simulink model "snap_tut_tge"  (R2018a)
settings: Solver=VariableStepDiscrete  StartTime=0.0  StopTime=50000  RelTol=1e-3
undefined symbols (not defined in the file): bad_frame, Bit, Both, bram, c, cnt_rst, core_rst, d, data, data_in, eof, eof_in, Falling, hex2dec, ip, ip_in, led, led_rx, led_tx, led_up, link_up, Location, Lower, Minimum_Area, notused, out, overrun, reg, Rising, ROACH2, sfp, SNAP, tx_full, tx_over, Unsigned, Upper, valid, valid_in, Width, xc7k160t
libraries: xbsIndex_r4 x1201, casper_library_misc x9, xps_library x5
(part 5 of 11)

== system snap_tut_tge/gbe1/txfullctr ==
  out_reg : Inport
  assert_reg : xbsIndex_r4/Assert  assert_type=on  type_source=Explicitly  gui_display_data_type=Fixed-point  arith_type=Unsigned  n_bits=32  bin_pt=0  preci_type=Single  exp_width=8  frac_width=24  assert_rate=off  rate_source=Explicitly  period=1  output_port=on  block_type=assert
  cast_gw : xbsIndex_r4/Convert  gui_display_data_type=Fixed-point  arith_type=Unsigned  n_bits=32  bin_pt=0  float_type=Single  exp_bits=8  fraction_bits=24  quantization=Truncate  overflow=Wrap  en=off  latency=1  pipeline=off  dbl_ovrd=off  block_type=convert
  io_delay : xbsIndex_r4/Delay  rst=off  infoeditControl=Selection of Reset will increase slice count due to use of real FFs and instead of SRLs  en=off  latency=1  reg_retiming=on  dbl_ovrd=off  block_type=delay
  reint1 : xbsIndex_r4/Reinterpret  force_arith_type=on  arith_type=Unsigned  force_bin_pt=on  bin_pt=0  block_type=reinterpret
  sim_out : Terminator
  snap_tut_tge_gbe1_txfullctr_user_data_in : xbsIndex_r4/Gateway Out  inherit_from_input=off  hdl_port=on  rows=1  columns=1  UseAsDAC=off  DACChannel='1'  interface=None  automatic_assignment=on  address_offset=hex2dec('00')  intf_name=''  intf_description=''  timing_constraint=None  locs_specified=off  LOCs={}  io_standard={}  block_type=gatewayout
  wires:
  io_delay/1 -> cast_gw/1
  cast_gw/1 -> snap_tut_tge_gbe1_txfullctr_user_data_in/1
  snap_tut_tge_gbe1_txfullctr_user_data_in/1 -> sim_out/1
  out_reg/1 -> assert_reg/1
  assert_reg/1 -> reint1/1
  reint1/1 -> io_delay/1

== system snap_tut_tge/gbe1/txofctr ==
  out_reg : Inport
  assert_reg : xbsIndex_r4/Assert  assert_type=on  type_source=Explicitly  gui_display_data_type=Fixed-point  arith_type=Unsigned  n_bits=32  bin_pt=0  preci_type=Single  exp_width=8  frac_width=24  assert_rate=off  rate_source=Explicitly  period=1  output_port=on  block_type=assert
  cast_gw : xbsIndex_r4/Convert  gui_display_data_type=Fixed-point  arith_type=Unsigned  n_bits=32  bin_pt=0  float_type=Single  exp_bits=8  fraction_bits=24  quantization=Truncate  overflow=Wrap  en=off  latency=1  pipeline=off  dbl_ovrd=off  block_type=convert
  io_delay : xbsIndex_r4/Delay  rst=off  infoeditControl=Selection of Reset will increase slice count due to use of real FFs and instead of SRLs  en=off  latency=1  reg_retiming=on  dbl_ovrd=off  block_type=delay
  reint1 : xbsIndex_r4/Reinterpret  force_arith_type=on  arith_type=Unsigned  force_bin_pt=on  bin_pt=0  block_type=reinterpret
  sim_out : Terminator
  snap_tut_tge_gbe1_txofctr_user_data_in : xbsIndex_r4/Gateway Out  inherit_from_input=off  hdl_port=on  rows=1  columns=1  UseAsDAC=off  DACChannel='1'  interface=None  automatic_assignment=on  address_offset=hex2dec('00')  intf_name=''  intf_description=''  timing_constraint=None  locs_specified=off  LOCs={}  io_standard={}  block_type=gatewayout
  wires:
  io_delay/1 -> cast_gw/1
  cast_gw/1 -> snap_tut_tge_gbe1_txofctr_user_data_in/1
  snap_tut_tge_gbe1_txofctr_user_data_in/1 -> sim_out/1
  out_reg/1 -> assert_reg/1
  assert_reg/1 -> reint1/1
  reint1/1 -> io_delay/1

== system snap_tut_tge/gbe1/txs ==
  in_link_up : Inport
  in_led_tx : Inport  Port=2
  in_tx_full : Inport  Port=3
  in_tx_over : Inport  Port=4
  in_valid : Inport  Port=5
  in_eof : Inport  Port=6
  in_data : Inport  Port=7
  in_ip : Inport  Port=8
  we : Inport  Port=9
  trig : Inport  Port=10
  assert_data : xbsIndex_r4/Assert  assert_type=on  type_source=Explicitly  gui_display_data_type=Fixed-point  arith_type=Unsigned  n_bits=64  bin_pt=0  preci_type=Single  exp_width=8  frac_width=24  assert_rate=off  rate_source=Explicitly  period=1  output_port=on  block_type=assert
  assert_eof : xbsIndex_r4/Assert  assert_type=on  type_source=Explicitly  gui_display_data_type=Boolean  arith_type=Boolean  n_bits=1  bin_pt=0  preci_type=Single  exp_width=8  frac_width=24  assert_rate=off  rate_source=Explicitly  period=1  output_port=on  block_type=assert
  assert_ip : xbsIndex_r4/Assert  assert_type=on  type_source=Explicitly  gui_display_data_type=Fixed-point  arith_type=Unsigned  n_bits=32  bin_pt=0  preci_type=Single  exp_width=8  frac_width=24  assert_rate=off  rate_source=Explicitly  period=1  output_port=on  block_type=assert
  assert_led_tx : xbsIndex_r4/Assert  assert_type=on  type_source=Explicitly  gui_display_data_type=Boolean  arith_type=Boolean  n_bits=1  bin_pt=0  preci_type=Single  exp_width=8  frac_width=24  assert_rate=off  rate_source=Explicitly  period=1  output_port=on  block_type=assert
  assert_link_up : xbsIndex_r4/Assert  assert_type=on  type_source=Explicitly  gui_display_data_type=Boolean  arith_type=Boolean  n_bits=1  bin_pt=0  preci_type=Single  exp_width=8  frac_width=24  assert_rate=off  rate_source=Explicitly  period=1  output_port=on  block_type=assert
  assert_tx_full : xbsIndex_r4/Assert  assert_type=on  type_source=Explicitly  gui_display_data_type=Boolean  arith_type=Boolean  n_bits=1  bin_pt=0  preci_type=Single  exp_width=8  frac_width=24  assert_rate=off  rate_source=Explicitly  period=1  output_port=on  block_type=assert
  assert_tx_over : xbsIndex_r4/Assert  assert_type=on  type_source=Explicitly  gui_display_data_type=Boolean  arith_type=Boolean  n_bits=1  bin_pt=0  preci_type=Single  exp_width=8  frac_width=24  assert_rate=off  rate_source=Explicitly  period=1  output_port=on  block_type=assert
  assert_valid : xbsIndex_r4/Assert  assert_type=on  type_source=Explicitly  gui_display_data_type=Boolean  arith_type=Boolean  n_bits=1  bin_pt=0  preci_type=Single  exp_width=8  frac_width=24  assert_rate=off  rate_source=Explicitly  period=1  output_port=on  block_type=assert
  buscreate : Subsystem  AncestorBlock=casper_library_flow_control/bus_create  mask(bus_create){inputNum=8}
      mask prompts: inputNum "Number of inputs:"
      mask init:
      | bus_create_init(gcb,...
      |     'inputNum', inputNum);
  io_delay : Subsystem  AncestorBlock=casper_library_delays/pipeline  mask(pipeline){csp_latency=5}
      mask prompts: csp_latency "Latency"
      mask help: An explicitly laid-out delay line to avoid mapping to SRL16s for use in pipelining to help achieve timing closure.
      mask init:
      | pipeline_init(gcb,'latency',csp_latency);
  ss : Subsystem  Tag=casper:snapshot  AncestorBlock=casper_library_scopes/snapshot  mask(snapshot){storage=bram, dram_dimm=2, dram_clock=250, nsamples=13, data_width=128, offset=off, circap=off, value=off, ext_arm=off, ext_circ=off, provide_outputs=off, use_dsp48=on}
      mask prompts: storage "Storage medium"; dram_dimm "DRAM dimm"; dram_clock "DRAM clock rate"; nsamples "Number of Samples (2^?)"; data_width "Data width"; offset "Start delay support"; circap "Circular capture support"; value "Extra value capture support"; ext_arm "External arm support"; ext_circ "External circular capture support"; provide_outputs "Provide outputs"; use_dsp48 "Use DSP48s to implement counters"
      mask help: Standard snap block, but with the following optional extras; 1) Optionally delay the fabric trigger by a user-specified number of valids. 2) Capture continuously after a trigger until a stop pulse is received. Data is captured into BRAM continuously, with old data being overwritten until a stop command is received. Then stop capturing when memory is filled. This enables you to get some data before and some data after the stop pulse. Use the 'tr_en_cnt' register to determine where you are in your vector. 'Addr' register's MSb now indicates 'busy capturing'. 3) Optionally capture a value on an i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
      mask init:
      | snapshot_init(gcb, ...
      |     'storage', storage, ...
      |     'dram_dimm', dram_dimm, ...
      |     'dram_clock', dram_clock, ...
      |     'nsamples', nsamples, ...
      |     'data_width', data_width, ...
      |     'offset', offset, ...
      |     'circap', circap, ...
      |     'value', value, ...
      |     'ext_arm', ext_arm, ...
      |     'ext_circ', ext_circ, ...
      |     'provide_outputs', 'off', ...
      |     'use_dsp48', use_dsp48);
  trig_delay : Subsystem  AncestorBlock=casper_library_delays/pipeline  mask(pipeline){csp_latency=5}
      mask prompts: csp_latency "Latency"
      mask help: An explicitly laid-out delay line to avoid mapping to SRL16s for use in pipelining to help achieve timing closure.
      mask init:
      | pipeline_init(gcb,'latency',csp_latency);
  we_delay : Subsystem  AncestorBlock=casper_library_delays/pipeline  mask(pipeline){csp_latency=5}
      mask prompts: csp_latency "Latency"
      mask help: An explicitly laid-out delay line to avoid mapping to SRL16s for use in pipelining to help achieve timing closure.
      mask init:
      | pipeline_init(gcb,'latency',csp_latency);
  arm_out : Outport
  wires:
  ss/1(arm_out) -> arm_out/1
  buscreate/1(bus_out) -> io_delay/1(d)
  io_delay/1(q) -> ss/1(din)
  in_link_up/1 -> assert_link_up/1
  assert_link_up/1 -> buscreate/1(in1)
  in_led_tx/1 -> assert_led_tx/1
  assert_led_tx/1 -> buscreate/2(in2)
  in_tx_full/1 -> assert_tx_full/1
  assert_tx_full/1 -> buscreate/3(in3)
  in_tx_over/1 -> assert_tx_over/1
  assert_tx_over/1 -> buscreate/4(in4)
  in_valid/1 -> assert_valid/1
  assert_valid/1 -> buscreate/5(in5)
  in_eof/1 -> assert_eof/1
  assert_eof/1 -> buscreate/6(in6)
  in_data/1 -> assert_data/1
  assert_data/1 -> buscreate/7(in7)
  in_ip/1 -> assert_ip/1
  assert_ip/1 -> buscreate/8(in8)
  we/1 -> we_delay/1(d)
  we_delay/1(q) -> ss/2(we)
  trig/1 -> trig_delay/1(d)
  trig_delay/1(q) -> ss/3(trig)

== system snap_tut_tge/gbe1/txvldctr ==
  out_reg : Inport
  assert_reg : xbsIndex_r4/Assert  assert_type=on  type_source=Explicitly  gui_display_data_type=Fixed-point  arith_type=Unsigned  n_bits=32  bin_pt=0  preci_type=Single  exp_width=8  frac_width=24  assert_rate=off  rate_source=Explicitly  period=1  output_port=on  block_type=assert
  cast_gw : xbsIndex_r4/Convert  gui_display_data_type=Fixed-point  arith_type=Unsigned  n_bits=32  bin_pt=0  float_type=Single  exp_bits=8  fraction_bits=24  quantization=Truncate  overflow=Wrap  en=off  latency=1  pipeline=off  dbl_ovrd=off  block_type=convert
  io_delay : xbsIndex_r4/Delay  rst=off  infoeditControl=Selection of Reset will increase slice count due to use of real FFs and instead of SRLs  en=off  latency=1  reg_retiming=on  dbl_ovrd=off  block_type=delay
  reint1 : xbsIndex_r4/Reinterpret  force_arith_type=on  arith_type=Unsigned  force_bin_pt=on  bin_pt=0  block_type=reinterpret
  sim_out : Terminator
  snap_tut_tge_gbe1_txvldctr_user_data_in : xbsIndex_r4/Gateway Out  inherit_from_input=off  hdl_port=on  rows=1  columns=1  UseAsDAC=off  DACChannel='1'  interface=None  automatic_assignment=on  address_offset=hex2dec('00')  intf_name=''  intf_description=''  timing_constraint=None  locs_specified=off  LOCs={}  io_standard={}  block_type=gatewayout
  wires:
  io_delay/1 -> cast_gw/1
  cast_gw/1 -> snap_tut_tge_gbe1_txvldctr_user_data_in/1
  snap_tut_tge_gbe1_txvldctr_user_data_in/1 -> sim_out/1
  out_reg/1 -> assert_reg/1
  assert_reg/1 -> reint1/1
  reint1/1 -> io_delay/1

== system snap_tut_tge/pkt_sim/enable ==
  sim_1 : Inport
  convert1_1 : DataTypeConversion  OutDataTypeStr=fixdt('ufix32_En0')
  convert2_1 : DataTypeConversion  OutDataTypeStr=fixdt('ufix32_En0')  ConvertRealWorld=Stored Integer (SI)
  gain_1 : Gain
  io_delay : xbsIndex_r4/Delay  rst=off  infoeditControl=Selection of Reset will increase slice count due to use of real FFs and instead of SRLs  en=off  latency=0  reg_retiming=on  dbl_ovrd=off  block_type=delay
  reint1 : xbsIndex_r4/Reinterpret  force_arith_type=on  arith_type=Unsigned  force_bin_pt=on  bin_pt=0  block_type=reinterpret
  slice_reg : xbsIndex_r4/Slice  nbits=32  boolean_output=off  mode=Lower Bit Location + Width  bit1=0  base1=MSB of Input  bit0=0  base0=LSB of Input  dbl_ovrd=off  block_type=slice
  snap_tut_tge_pkt_sim_enable_user_data_out : xbsIndex_r4/Gateway In  gui_display_data_type=Fixed-point  arith_type=Unsigned  n_bits=32  bin_pt=0  preci_type=Single  exp_width=8  frac_width=24  rows=1  columns=1  quantization="Round  (unbiased: +/- Inf)"  overflow=Saturate  period=1  UseAsADC=off  ADCChannel='1'  interface=None  automatic_assignment=on  address_offset=hex2dec('00')  intf_name=''  intf_description=''  default_value=0  timing_constraint=None  locs_specified=off  LOCs={}  io_standard={}  inherit_from_input=off  hdl_port=on  dbl_ovrd=off  block_type=gatewayin
  in_reg : Outport
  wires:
  snap_tut_tge_pkt_sim_enable_user_data_out/1 -> io_delay/1
  sim_1/1 -> convert1_1/1
  convert1_1/1 -> convert2_1/1
  convert2_1/1 -> gain_1/1
  gain_1/1 -> snap_tut_tge_pkt_sim_enable_user_data_out/1
  io_delay/1 -> slice_reg/1
  slice_reg/1 -> reint1/1
  reint1/1 -> in_reg/1

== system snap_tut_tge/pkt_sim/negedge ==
  in : Inport
  Delay : xbsIndex_r4/Delay  rst=off  infoeditControl=Selection of Reset will increase slice count due to use of real FFs and instead of SRLs  en=off  latency=1  reg_retiming=off  dbl_ovrd=off  block_type=delay
  Inverter : xbsIndex_r4/Inverter  en=off  latency=0  dbl_ovrd=off  block_type=inv
  edge_op : xbsIndex_r4/Logical  logical_function=AND  inputs=2  en=off  latency=0  precision=Full  arith_type=Unsigned  n_bits=8  bin_pt=2  align_bp=on  dbl_ovrd=off  block_type=logical
  out : Outport
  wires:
  Inverter/1 -> edge_op/1
  edge_op/1 -> out/1
  in/1 -> Inverter/1, Delay/1
  Delay/1 -> edge_op/2

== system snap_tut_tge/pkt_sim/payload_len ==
  sim_1 : Inport
  convert1_1 : DataTypeConversion  OutDataTypeStr=fixdt('ufix32_En0')
  convert2_1 : DataTypeConversion  OutDataTypeStr=fixdt('ufix32_En0')  ConvertRealWorld=Stored Integer (SI)
  gain_1 : Gain
  io_delay : xbsIndex_r4/Delay  rst=off  infoeditControl=Selection of Reset will increase slice count due to use of real FFs and instead of SRLs  en=off  latency=0  reg_retiming=on  dbl_ovrd=off  block_type=delay
  reint1 : xbsIndex_r4/Reinterpret  force_arith_type=on  arith_type=Unsigned  force_bin_pt=on  bin_pt=0  block_type=reinterpret
  slice_reg : xbsIndex_r4/Slice  nbits=32  boolean_output=off  mode=Lower Bit Location + Width  bit1=0  base1=MSB of Input  bit0=0  base0=LSB of Input  dbl_ovrd=off  block_type=slice
  snap_tut_tge_pkt_sim_payload_len_user_data_out : xbsIndex_r4/Gateway In  gui_display_data_type=Fixed-point  arith_type=Unsigned  n_bits=32  bin_pt=0  preci_type=Single  exp_width=8  frac_width=24  rows=1  columns=1  quantization="Round  (unbiased: +/- Inf)"  overflow=Saturate  period=1  UseAsADC=off  ADCChannel='1'  interface=None  automatic_assignment=on  address_offset=hex2dec('00')  intf_name=''  intf_description=''  default_value=0  timing_constraint=None  locs_specified=off  LOCs={}  io_standard={}  inherit_from_input=off  hdl_port=on  dbl_ovrd=off  block_type=gatewayin
  in_reg : Outport
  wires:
  snap_tut_tge_pkt_sim_payload_len_user_data_out/1 -> io_delay/1
  sim_1/1 -> convert1_1/1
  convert1_1/1 -> convert2_1/1
  convert2_1/1 -> gain_1/1
  gain_1/1 -> snap_tut_tge_pkt_sim_payload_len_user_data_out/1
  io_delay/1 -> slice_reg/1
  slice_reg/1 -> reint1/1
  reint1/1 -> in_reg/1

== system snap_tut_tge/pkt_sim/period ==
  sim_1 : Inport
  convert1_1 : DataTypeConversion  OutDataTypeStr=fixdt('ufix32_En0')
  convert2_1 : DataTypeConversion  OutDataTypeStr=fixdt('ufix32_En0')  ConvertRealWorld=Stored Integer (SI)
  gain_1 : Gain
  io_delay : xbsIndex_r4/Delay  rst=off  infoeditControl=Selection of Reset will increase slice count due to use of real FFs and instead of SRLs  en=off  latency=0  reg_retiming=on  dbl_ovrd=off  block_type=delay
  reint1 : xbsIndex_r4/Reinterpret  force_arith_type=on  arith_type=Unsigned  force_bin_pt=on  bin_pt=0  block_type=reinterpret
  slice_reg : xbsIndex_r4/Slice  nbits=32  boolean_output=off  mode=Lower Bit Location + Width  bit1=0  base1=MSB of Input  bit0=0  base0=LSB of Input  dbl_ovrd=off  block_type=slice
  snap_tut_tge_pkt_sim_period_user_data_out : xbsIndex_r4/Gateway In  gui_display_data_type=Fixed-point  arith_type=Unsigned  n_bits=32  bin_pt=0  preci_type=Single  exp_width=8  frac_width=24  rows=1  columns=1  quantization="Round  (unbiased: +/- Inf)"  overflow=Saturate  period=1  UseAsADC=off  ADCChannel='1'  interface=None  automatic_assignment=on  address_offset=hex2dec('00')  intf_name=''  intf_description=''  default_value=0  timing_constraint=None  locs_specified=off  LOCs={}  io_standard={}  inherit_from_input=off  hdl_port=on  dbl_ovrd=off  block_type=gatewayin
  in_reg : Outport
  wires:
  snap_tut_tge_pkt_sim_period_user_data_out/1 -> io_delay/1
  sim_1/1 -> convert1_1/1
  convert1_1/1 -> convert2_1/1
  convert2_1/1 -> gain_1/1
  gain_1/1 -> snap_tut_tge_pkt_sim_period_user_data_out/1
  io_delay/1 -> slice_reg/1
  slice_reg/1 -> reint1/1
  reint1/1 -> in_reg/1

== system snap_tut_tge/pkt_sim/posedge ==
  in : Inport
  Delay : xbsIndex_r4/Delay  rst=off  infoeditControl=Selection of Reset will increase slice count due to use of real FFs and instead of SRLs  en=off  latency=1  reg_retiming=off  dbl_ovrd=off  block_type=delay
  Inverter : xbsIndex_r4/Inverter  en=off  latency=0  dbl_ovrd=off  block_type=inv
  edge_op : xbsIndex_r4/Logical  logical_function=NOR  inputs=2  en=off  latency=0  precision=Full  arith_type=Unsigned  n_bits=8  bin_pt=2  align_bp=on  dbl_ovrd=off  block_type=logical
  out : Outport
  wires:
  Inverter/1 -> edge_op/1
  edge_op/1 -> out/1
  in/1 -> Inverter/1, Delay/1
  Delay/1 -> edge_op/2

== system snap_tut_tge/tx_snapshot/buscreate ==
  in1 : Inport
  in2 : Inport  Port=2
  in3 : Inport  Port=3
  concatenate : xbsIndex_r4/Concat  num_inputs=3  dbl_ovrd=off  block_type=concat
  reinterpret1 : xbsIndex_r4/Reinterpret  force_arith_type=on  arith_type=Unsigned  force_bin_pt=on  bin_pt=0  block_type=reinterpret
  reinterpret2 : xbsIndex_r4/Reinterpret  force_arith_type=on  arith_type=Unsigned  force_bin_pt=on  bin_pt=0  block_type=reinterpret
  reinterpret3 : xbsIndex_r4/Reinterpret  force_arith_type=on  arith_type=Unsigned  force_bin_pt=on  bin_pt=0  block_type=reinterpret
  bus_out : Outport
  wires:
  concatenate/1 -> bus_out/1
  in1/1 -> reinterpret1/1
  reinterpret1/1 -> concatenate/1
  in2/1 -> reinterpret2/1
  reinterpret2/1 -> concatenate/2
  in3/1 -> reinterpret3/1
  reinterpret3/1 -> concatenate/3

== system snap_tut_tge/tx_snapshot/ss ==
  note: Generate stop when in circular capture mode
  note: Delay start of capture
  note: ctrl: bit0: Put a posedge here to enable a new capture. bit1: ignore external trigger and trigger immediately. bit2: ignore external write enable and capture on every FPGA clock. bit3: continuously capture data until we get an external stop command.
  note: Offset in vector from first element captured, used during circular capture
  note: Number of bytes in buffer and done bit
  note: Number of valid data samples to skip after trigger before starting capture
  note: Value on vin aligned with first sample on din captured
  din : Inport
  we : Inport  Port=2
  trig : Inport  Port=3
  add_del : xbsIndex_r4/Delay  rst=off  infoeditControl=Selection of Reset will increase slice count due to use of real FFs and instead of SRLs  en=off  latency=1  reg_retiming=on  dbl_ovrd=off  block_type=delay
  add_gen : Subsystem  AncestorBlock=casper_library_scopes/snapshot/add_gen  mask{counter_size=12+4+1, increment=16, nsamples=12, burst_size=0, use_dsp48=on}
      mask prompts: counter_size "Address counter size (2^?)"; increment "Address counter increment"; nsamples "Number of samples (2^?)"; burst_size "Burst size (2^?)"; use_dsp48 "dsp48 counter/s"
      mask init:
      | set_param(gcb,'LinkStatus','inactive');
      | if strcmp(use_dsp48,'on'),
      |     set_param([gcb,'/add_gen'],'implementation','DSP48');
      | else
      |     set_param([gcb,'/add_gen'],'implementation','Fabric');
      | end
  arm : xbsIndex_r4/Constant  const=0  gui_display_data_type=Fixed-point  arith_type=Boolean  n_bits=16  bin_pt=14  preci_type=Single  exp_width=8  frac_width=24  explicit_period=on  period=1  equ=P=C  opselect=C  inp2=PCIN>>17  opr=+  inp1=P  carry=CIN  dbl_ovrd=off  block_type=constant
  arm_or : xbsIndex_r4/Logical  logical_function=OR  inputs=2  en=off  latency=0  precision=Full  arith_type=Unsigned  n_bits=16  bin_pt=0  align_bp=on  dbl_ovrd=off  block_type=logical
  basic_ctrl : Subsystem  AncestorBlock=casper_library_scopes/snapshot/basic_ctrl  mask{dram=off, data_width=128}
      mask prompts: data_width "data width"
      mask init:
      | set_param(gcb,'LinkStatus','inactive');
      | set_param([gcb,'/dram_munge'], 'dram', dram);
  bram : Subsystem  Tag=xps:bram  AncestorBlock=xps_library/Memory/shared_bram  mask{arith_type=Unsigned, addr_width=12, data_width=128, reg_prim_output=off, reg_core_output=off, optimization=Minimum_Area, data_bin_pt=0, init_vals=[0:2^12-1], sample_rate=1}
      mask prompts: arith_type "Output Data Type"; addr_width "Address width"; data_width "Data Width"; reg_prim_output "Register Primitive Output"; reg_core_output "Register Core Output"; data_bin_pt "Data Binary Point"; init_vals "Initial values (simulation only)"; sample_rate "Sample rate"
      mask init:
      | shared_bram_mask;
  cast : xbsIndex_r4/Convert  gui_display_data_type=Fixed-point  arith_type=Unsigned  n_bits=128  bin_pt=0  float_type=Single  exp_bits=8  fraction_bits=24  quantization=Truncate  overflow=Wrap  en=off  latency=0  pipeline=off  dbl_ovrd=off  block_type=convert
  circ : xbsIndex_r4/Constant  const=0  gui_display_data_type=Fixed-point  arith_type=Boolean  n_bits=16  bin_pt=14  preci_type=Single  exp_width=8  frac_width=24  explicit_period=on  period=1  equ=P=C  opselect=C  inp2=PCIN>>17  opr=+  inp1=P  carry=CIN  dbl_ovrd=off  block_type=constant
  circ_or : xbsIndex_r4/Logical  logical_function=OR  inputs=2  en=off  latency=0  precision=Full  arith_type=Unsigned  n_bits=16  bin_pt=0  align_bp=on  dbl_ovrd=off  block_type=logical
  ctrl : Subsystem  Tag=xps:sw_reg  AncestorBlock=xps_library/Memory/software_register  mask(swreg){io_dir=From Processor, io_delay=0, init_val=0, sample_period=1, names=reg, bitwidths=32, bin_pts=0, arith_types=0, sim_port=off, show_format=on}
      mask prompts: io_dir "I/O direction"; io_delay "I/O delay"; init_val "Initial Value"; sample_period "Sample period"; names "Bitfield names [msb...lsb]"; bitwidths "Bitfield widths"; bin_pts "Bitfield binary pts"; arith_types "Bitfield types, ufix=0, fix=1, bool=2"; sim_port "Provide sim input/output?"; show_format "Print format string?"
      mask help: A 32-bit software-accessible register. Can be divided into bitfields of varying widths and types using the fields in the block mask.
      mask init:
      | swreg_init(gcb)
  ctrl_combine : Subsystem  AncestorBlock=casper_library_flow_control/bus_create  mask(bus_create){inputNum=4}
      mask prompts: inputNum "Number of inputs:"
      mask init:
      | bus_create_init(gcb,...
      |     'inputNum', inputNum);
  ctrl_split : Subsystem  AncestorBlock=casper_library_flow_control/bus_expand  mask(bus_expand){mode=divisions of arbitrary size, outputNum=1, outputWidth=[28 1 2 1], outputBinaryPt=0, outputArithmeticType=[0 2 0 2], show_format=on, outputToWorkspace=off, variablePrefix=out, outputToModelAsWell=on}
      mask prompts: outputNum "Number of outputs:"; outputWidth "Output width [msb ... lsb]:"; outputBinaryPt "Output binary point position [msb ... lsb]:"; outputArithmeticType "Output arithmetic type (ufix=0, fix=1, bool=2) [msb ... lsb]:"; show_format "Print format string?"; outputToWorkspace "Output to workspace?"; variablePrefix "Variable name prefix:"; outputToModelAsWell "Output to model as well?"
      mask help: Expands a 'bus' made using a bus_create or Xilinx concat block. The input will be divided into the specified number of outputs with the specified arithmetic types. Divisions are made from most significant bit.
      mask init:
      | bus_expand_init(gcb,...
      |     'mode', mode, ...
      |     'outputNum', outputNum, ...
      |     'outputWidth', outputWidth, ...
      |     'outputBinaryPt', outputBinaryPt, ...
      |     'outputArithmeticType', outputArithmeticType, ...
      |     'show_format', show_format, ...
      |     'outputToWorkspace', outputToWorkspace, ...
      |     'variablePrefix', variablePrefix, ...
      |     'outputToModelAsWell', outputToModelAsWell);
  dat_del : xbsIndex_r4/Delay  rst=off  infoeditControl=Selection of Reset will increase slice count due to use of real FFs and instead of SRLs  en=off  latency=1  reg_retiming=on  dbl_ovrd=off  block_type=delay
  g_tr_en_cnt : Terminator
  gbram : Terminator
  goto_ss_we2_const : xbsIndex_r4/Constant  const=0  gui_display_data_type=Fixed-point  arith_type=Boolean  n_bits=16  bin_pt=14  preci_type=Single  exp_width=8  frac_width=24  explicit_period=on  period=1  equ=P=C  opselect=C  inp2=PCIN>>17  opr=+  inp1=P  carry=CIN  dbl_ovrd=off  block_type=constant
  goto_ss_we3_const : xbsIndex_r4/Constant  const=0  gui_display_data_type=Fixed-point  arith_type=Boolean  n_bits=16  bin_pt=14  preci_type=Single  exp_width=8  frac_width=24  explicit_period=on  period=1  equ=P=C  opselect=C  inp2=PCIN>>17  opr=+  inp1=P  carry=CIN  dbl_ovrd=off  block_type=constant
  gval : Terminator
  never : xbsIndex_r4/Constant  const=0  gui_display_data_type=Fixed-point  arith_type=Boolean  n_bits=16  bin_pt=14  preci_type=Single  exp_width=8  frac_width=24  explicit_period=on  period=1  equ=P=C  opselect=C  inp2=PCIN>>17  opr=+  inp1=P  carry=CIN  dbl_ovrd=off  block_type=constant
  ri : xbsIndex_r4/Reinterpret  force_arith_type=on  arith_type=Unsigned  force_bin_pt=on  bin_pt=0  block_type=reinterpret
  status : Subsystem  Tag=xps:sw_reg  AncestorBlock=xps_library/Memory/software_register  mask(swreg){io_dir=To Processor, io_delay=0, init_val=0, sample_period=1, names=reg, bitwidths=32, bin_pts=0, arith_types=0, sim_port=off, show_format=on}
      mask prompts: io_dir "I/O direction"; io_delay "I/O delay"; init_val "Initial Value"; sample_period "Sample period"; names "Bitfield names [msb...lsb]"; bitwidths "Bitfield widths"; bin_pts "Bitfield binary pts"; arith_types "Bitfield types, ufix=0, fix=1, bool=2"; sim_port "Provide sim input/output?"; show_format "Print format string?"
      mask help: A 32-bit software-accessible register. Can be divided into bitfields of varying widths and types using the fields in the block mask.
      mask init:
      | swreg_init(gcb)
  vin_const : xbsIndex_r4/Constant  const=0  gui_display_data_type=Fixed-point  arith_type=Boolean  n_bits=16  bin_pt=14  preci_type=Single  exp_width=8  frac_width=24  explicit_period=on  period=1  equ=P=C  opselect=C  inp2=PCIN>>17  opr=+  inp1=P  carry=CIN  dbl_ovrd=off  block_type=constant
  we_del : xbsIndex_r4/Delay  rst=off  infoeditControl=Selection of Reset will increase slice count due to use of real FFs and instead of SRLs  en=off  latency=1  reg_retiming=on  dbl_ovrd=off  block_type=delay
  arm_out : Outport
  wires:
  din/1 -> ri/1
  ri/1 -> cast/1
  cast/1 -> basic_ctrl/2(din)
  we/1 -> basic_ctrl/3(we)
  trig/1 -> basic_ctrl/4(trig)
  ctrl_combine/1(bus_out) -> basic_ctrl/5(ctrl)
  never/1 -> basic_ctrl/6(stopi)
  arm/1 -> arm_or/2
  arm_or/1 -> arm_out/1, ctrl_combine/4(in4)
  circ/1 -> circ_or/2
  ctrl/1(in_reg) -> ctrl_split/1(bus_in)
  ctrl_split/1(msb_out4) -> ctrl_combine/1(in1)
  ctrl_split/2(out3) -> circ_or/1
  ctrl_split/3(out2) -> ctrl_combine/3(in3)
  ctrl_split/4(lsb_out1) -> arm_or/1
  circ_or/1 -> ctrl_combine/2(in2)
  basic_ctrl/1(vout) -> add_gen/1(vin)
  basic_ctrl/2(dout) -> add_gen/2(din)
  basic_ctrl/3(we_o) -> add_gen/3(we), [goto_48692828_we1]
  basic_ctrl/4(go) -> add_gen/4(go)
  basic_ctrl/5(stop) -> add_gen/5(cont)
  basic_ctrl/6(init) -> add_gen/6(init)
  add_gen/5(status) -> status/1(out_reg)
  vin_const/1 -> basic_ctrl/1(vin)
  add_gen/1(vout) -> gval/1
  add_gen/6(en_cnt) -> g_tr_en_cnt/1
  add_gen/2(add) -> add_del/1
  add_gen/3(dout) -> dat_del/1
  add_gen/4(we_o) -> we_del/1, [goto_48692828_we4]
  add_del/1 -> bram/1(addr)
  dat_del/1 -> bram/2(data_in)
  we_del/1 -> bram/3(we)
  bram/1(data_out) -> gbram/1
  goto_ss_we2_const/1 -> [goto_48692828_we2]
  goto_ss_we3_const/1 -> [goto_48692828_we3]

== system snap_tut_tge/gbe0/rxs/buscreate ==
  in1 : Inport
  in2 : Inport  Port=2
  in3 : Inport  Port=3
  in4 : Inport  Port=4
  in5 : Inport  Port=5
  in6 : Inport  Port=6
  in7 : Inport  Port=7
  in8 : Inport  Port=8
  concatenate : xbsIndex_r4/Concat  num_inputs=8  dbl_ovrd=off  block_type=concat
  reinterpret{1..8} (8 alike) : xbsIndex_r4/Reinterpret  force_arith_type=on  arith_type=Unsigned  force_bin_pt=on  bin_pt=0  block_type=reinterpret
  bus_out : Outport
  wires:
  concatenate/1 -> bus_out/1
  in1/1 -> reinterpret1/1
  reinterpret1/1 -> concatenate/1
  in2/1 -> reinterpret2/1
  reinterpret2/1 -> concatenate/2
  in3/1 -> reinterpret3/1
  reinterpret3/1 -> concatenate/3
  in4/1 -> reinterpret4/1
  reinterpret4/1 -> concatenate/4
  in5/1 -> reinterpret5/1
  reinterpret5/1 -> concatenate/5
  in6/1 -> reinterpret6/1
  reinterpret6/1 -> concatenate/6
  in7/1 -> reinterpret7/1
  reinterpret7/1 -> concatenate/7
  in8/1 -> reinterpret8/1
  reinterpret8/1 -> concatenate/8

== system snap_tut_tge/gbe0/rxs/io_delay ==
  d : Inport
  Register{0..4} (5 alike) : xbsIndex_r4/Register  init=0  rst=off  en=off  dbl_ovrd=off  block_type=register
  q : Outport
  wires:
  Register0/1 -> Register1/1
  Register1/1 -> Register2/1
  Register2/1 -> Register3/1
  Register3/1 -> Register4/1
  d/1 -> Register0/1
  Register4/1 -> q/1

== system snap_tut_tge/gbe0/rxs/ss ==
  note: Generate stop when in circular capture mode
  note: Delay start of capture
  note: ctrl: bit0: Put a posedge here to enable a new capture. bit1: ignore external trigger and trigger immediately. bit2: ignore external write enable and capture on every FPGA clock. bit3: continuously capture data until we get an external stop command.
  note: Offset in vector from first element captured, used during circular capture
  note: Number of bytes in buffer and done bit
  note: Number of valid data samples to skip after trigger before starting capture
  note: Value on vin aligned with first sample on din captured
  din : Inport
  we : Inport  Port=2
  trig : Inport  Port=3
  add_del : xbsIndex_r4/Delay  rst=off  infoeditControl=Selection of Reset will increase slice count due to use of real FFs and instead of SRLs  en=off  latency=1  reg_retiming=on  dbl_ovrd=off  block_type=delay
  add_gen : Subsystem  AncestorBlock=casper_library_scopes/snapshot/add_gen  mask{counter_size=13+4+1, increment=16, nsamples=13, burst_size=0, use_dsp48=on}
      mask prompts: counter_size "Address counter size (2^?)"; increment "Address counter increment"; nsamples "Number of samples (2^?)"; burst_size "Burst size (2^?)"; use_dsp48 "dsp48 counter/s"
      mask init:
      | set_param(gcb,'LinkStatus','inactive');
      | if strcmp(use_dsp48,'on'),
      |     set_param([gcb,'/add_gen'],'implementation','DSP48');
      | else
      |     set_param([gcb,'/add_gen'],'implementation','Fabric');
      | end
  arm : xbsIndex_r4/Constant  const=0  gui_display_data_type=Fixed-point  arith_type=Boolean  n_bits=16  bin_pt=14  preci_type=Single  exp_width=8  frac_width=24  explicit_period=on  period=1  equ=P=C  opselect=C  inp2=PCIN>>17  opr=+  inp1=P  carry=CIN  dbl_ovrd=off  block_type=constant
  arm_or : xbsIndex_r4/Logical  logical_function=OR  inputs=2  en=off  latency=0  precision=Full  arith_type=Unsigned  n_bits=16  bin_pt=0  align_bp=on  dbl_ovrd=off  block_type=logical
  basic_ctrl : Subsystem  AncestorBlock=casper_library_scopes/snapshot/basic_ctrl  mask{dram=off, data_width=128}
      mask prompts: data_width "data width"
      mask init:
      | set_param(gcb,'LinkStatus','inactive');
      | set_param([gcb,'/dram_munge'], 'dram', dram);
  bram : Subsystem  Tag=xps:bram  AncestorBlock=xps_library/Memory/shared_bram  mask{arith_type=Unsigned, addr_width=13, data_width=128, reg_prim_output=off, reg_core_output=off, optimization=Minimum_Area, data_bin_pt=0, init_vals=[0:2^13-1], sample_rate=1}
      mask prompts: arith_type "Output Data Type"; addr_width "Address width"; data_width "Data Width"; reg_prim_output "Register Primitive Output"; reg_core_output "Register Core Output"; data_bin_pt "Data Binary Point"; init_vals "Initial values (simulation only)"; sample_rate "Sample rate"
      mask init:
      | shared_bram_mask;
  cast : xbsIndex_r4/Convert  gui_display_data_type=Fixed-point  arith_type=Unsigned  n_bits=128  bin_pt=0  float_type=Single  exp_bits=8  fraction_bits=24  quantization=Truncate  overflow=Wrap  en=off  latency=0  pipeline=off  dbl_ovrd=off  block_type=convert
  circ : xbsIndex_r4/Constant  const=0  gui_display_data_type=Fixed-point  arith_type=Boolean  n_bits=16  bin_pt=14  preci_type=Single  exp_width=8  frac_width=24  explicit_period=on  period=1  equ=P=C  opselect=C  inp2=PCIN>>17  opr=+  inp1=P  carry=CIN  dbl_ovrd=off  block_type=constant
  circ_or : xbsIndex_r4/Logical  logical_function=OR  inputs=2  en=off  latency=0  precision=Full  arith_type=Unsigned  n_bits=16  bin_pt=0  align_bp=on  dbl_ovrd=off  block_type=logical
  ctrl : Subsystem  Tag=xps:sw_reg  AncestorBlock=xps_library/Memory/software_register  mask(swreg){io_dir=From Processor, io_delay=0, init_val=0, sample_period=1, names=reg, bitwidths=32, bin_pts=0, arith_types=0, sim_port=off, show_format=on}
      mask prompts: io_dir "I/O direction"; io_delay "I/O delay"; init_val "Initial Value"; sample_period "Sample period"; names "Bitfield names [msb...lsb]"; bitwidths "Bitfield widths"; bin_pts "Bitfield binary pts"; arith_types "Bitfield types, ufix=0, fix=1, bool=2"; sim_port "Provide sim input/output?"; show_format "Print format string?"
      mask help: A 32-bit software-accessible register. Can be divided into bitfields of varying widths and types using the fields in the block mask.
      mask init:
      | swreg_init(gcb)
  ctrl_combine : Subsystem  AncestorBlock=casper_library_flow_control/bus_create  mask(bus_create){inputNum=4}
      mask prompts: inputNum "Number of inputs:"
      mask init:
      | bus_create_init(gcb,...
      |     'inputNum', inputNum);
  ctrl_split : Subsystem  AncestorBlock=casper_library_flow_control/bus_expand  mask(bus_expand){mode=divisions of arbitrary size, outputNum=1, outputWidth=[28 1 2 1], outputBinaryPt=0, outputArithmeticType=[0 2 0 2], show_format=on, outputToWorkspace=off, variablePrefix=out, outputToModelAsWell=on}
      mask prompts: outputNum "Number of outputs:"; outputWidth "Output width [msb ... lsb]:"; outputBinaryPt "Output binary point position [msb ... lsb]:"; outputArithmeticType "Output arithmetic type (ufix=0, fix=1, bool=2) [msb ... lsb]:"; show_format "Print format string?"; outputToWorkspace "Output to workspace?"; variablePrefix "Variable name prefix:"; outputToModelAsWell "Output to model as well?"
      mask help: Expands a 'bus' made using a bus_create or Xilinx concat block. The input will be divided into the specified number of outputs with the specified arithmetic types. Divisions are made from most significant bit.
      mask init:
      | bus_expand_init(gcb,...
      |     'mode', mode, ...
      |     'outputNum', outputNum, ...
      |     'outputWidth', outputWidth, ...
      |     'outputBinaryPt', outputBinaryPt, ...
      |     'outputArithmeticType', outputArithmeticType, ...
      |     'show_format', show_format, ...
      |     'outputToWorkspace', outputToWorkspace, ...
      |     'variablePrefix', variablePrefix, ...
      |     'outputToModelAsWell', outputToModelAsWell);
  dat_del : xbsIndex_r4/Delay  rst=off  infoeditControl=Selection of Reset will increase slice count due to use of real FFs and instead of SRLs  en=off  latency=1  reg_retiming=on  dbl_ovrd=off  block_type=delay
  g_tr_en_cnt : Terminator
  gbram : Terminator
  goto_ss_we2_const : xbsIndex_r4/Constant  const=0  gui_display_data_type=Fixed-point  arith_type=Boolean  n_bits=16  bin_pt=14  preci_type=Single  exp_width=8  frac_width=24  explicit_period=on  period=1  equ=P=C  opselect=C  inp2=PCIN>>17  opr=+  inp1=P  carry=CIN  dbl_ovrd=off  block_type=constant
  goto_ss_we3_const : xbsIndex_r4/Constant  const=0  gui_display_data_type=Fixed-point  arith_type=Boolean  n_bits=16  bin_pt=14  preci_type=Single  exp_width=8  frac_width=24  explicit_period=on  period=1  equ=P=C  opselect=C  inp2=PCIN>>17  opr=+  inp1=P  carry=CIN  dbl_ovrd=off  block_type=constant
  gval : Terminator
  never : xbsIndex_r4/Constant  const=0  gui_display_data_type=Fixed-point  arith_type=Boolean  n_bits=16  bin_pt=14  preci_type=Single  exp_width=8  frac_width=24  explicit_period=on  period=1  equ=P=C  opselect=C  inp2=PCIN>>17  opr=+  inp1=P  carry=CIN  dbl_ovrd=off  block_type=constant
  ri : xbsIndex_r4/Reinterpret  force_arith_type=on  arith_type=Unsigned  force_bin_pt=on  bin_pt=0  block_type=reinterpret
  status : Subsystem  Tag=xps:sw_reg  AncestorBlock=xps_library/Memory/software_register  mask(swreg){io_dir=To Processor, io_delay=0, init_val=0, sample_period=1, names=reg, bitwidths=32, bin_pts=0, arith_types=0, sim_port=off, show_format=on}
      mask prompts: io_dir "I/O direction"; io_delay "I/O delay"; init_val "Initial Value"; sample_period "Sample period"; names "Bitfield names [msb...lsb]"; bitwidths "Bitfield widths"; bin_pts "Bitfield binary pts"; arith_types "Bitfield types, ufix=0, fix=1, bool=2"; sim_port "Provide sim input/output?"; show_format "Print format string?"
      mask help: A 32-bit software-accessible register. Can be divided into bitfields of varying widths and types using the fields in the block mask.
      mask init:
      | swreg_init(gcb)
  vin_const : xbsIndex_r4/Constant  const=0  gui_display_data_type=Fixed-point  arith_type=Boolean  n_bits=16  bin_pt=14  preci_type=Single  exp_width=8  frac_width=24  explicit_period=on  period=1  equ=P=C  opselect=C  inp2=PCIN>>17  opr=+  inp1=P  carry=CIN  dbl_ovrd=off  block_type=constant
  we_del : xbsIndex_r4/Delay  rst=off  infoeditControl=Selection of Reset will increase slice count due to use of real FFs and instead of SRLs  en=off  latency=1  reg_retiming=on  dbl_ovrd=off  block_type=delay
  arm_out : Outport
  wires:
  din/1 -> ri/1
  ri/1 -> cast/1
  cast/1 -> basic_ctrl/2(din)
  we/1 -> basic_ctrl/3(we)
  trig/1 -> basic_ctrl/4(trig)
  ctrl_combine/1(bus_out) -> basic_ctrl/5(ctrl)
  never/1 -> basic_ctrl/6(stopi)
  arm/1 -> arm_or/2
  arm_or/1 -> arm_out/1, ctrl_combine/4(in4)
  circ/1 -> circ_or/2
  ctrl/1(in_reg) -> ctrl_split/1(bus_in)
  ctrl_split/1(msb_out4) -> ctrl_combine/1(in1)
  ctrl_split/2(out3) -> circ_or/1
  ctrl_split/3(out2) -> ctrl_combine/3(in3)
  ctrl_split/4(lsb_out1) -> arm_or/1
  circ_or/1 -> ctrl_combine/2(in2)
  basic_ctrl/1(vout) -> add_gen/1(vin)
  basic_ctrl/2(dout) -> add_gen/2(din)
  basic_ctrl/3(we_o) -> add_gen/3(we), [goto_23361247_we1]
  basic_ctrl/4(go) -> add_gen/4(go)
  basic_ctrl/5(stop) -> add_gen/5(cont)
  basic_ctrl/6(init) -> add_gen/6(init)
  add_gen/5(status) -> status/1(out_reg)
  vin_const/1 -> basic_ctrl/1(vin)
  add_gen/1(vout) -> gval/1
  add_gen/6(en_cnt) -> g_tr_en_cnt/1
  add_gen/2(add) -> add_del/1
  add_gen/3(dout) -> dat_del/1
  add_gen/4(we_o) -> we_del/1, [goto_23361247_we4]
  add_del/1 -> bram/1(addr)
  dat_del/1 -> bram/2(data_in)
  we_del/1 -> bram/3(we)
  bram/1(data_out) -> gbram/1
  goto_ss_we2_const/1 -> [goto_23361247_we2]
  goto_ss_we3_const/1 -> [goto_23361247_we3]

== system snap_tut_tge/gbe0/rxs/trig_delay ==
  d : Inport
  Register{0..4} (5 alike) : xbsIndex_r4/Register  init=0  rst=off  en=off  dbl_ovrd=off  block_type=register
  q : Outport
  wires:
  Register0/1 -> Register1/1
  Register1/1 -> Register2/1
  Register2/1 -> Register3/1
  Register3/1 -> Register4/1
  d/1 -> Register0/1
  Register4/1 -> q/1

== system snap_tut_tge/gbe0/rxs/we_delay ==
  d : Inport
  Register{0..4} (5 alike) : xbsIndex_r4/Register  init=0  rst=off  en=off  dbl_ovrd=off  block_type=register
  q : Outport
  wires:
  Register0/1 -> Register1/1
  Register1/1 -> Register2/1
  Register2/1 -> Register3/1
  Register3/1 -> Register4/1
  d/1 -> Register0/1
  Register4/1 -> q/1

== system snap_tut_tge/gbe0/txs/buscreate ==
  in1 : Inport
  in2 : Inport  Port=2
  in3 : Inport  Port=3
  in4 : Inport  Port=4
  in5 : Inport  Port=5
  in6 : Inport  Port=6
  in7 : Inport  Port=7
  in8 : Inport  Port=8
  concatenate : xbsIndex_r4/Concat  num_inputs=8  dbl_ovrd=off  block_type=concat
  reinterpret{1..8} (8 alike) : xbsIndex_r4/Reinterpret  force_arith_type=on  arith_type=Unsigned  force_bin_pt=on  bin_pt=0  block_type=reinterpret
  bus_out : Outport
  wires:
  concatenate/1 -> bus_out/1
  in1/1 -> reinterpret1/1
  reinterpret1/1 -> concatenate/1
  in2/1 -> reinterpret2/1
  reinterpret2/1 -> concatenate/2
  in3/1 -> reinterpret3/1
  reinterpret3/1 -> concatenate/3
  in4/1 -> reinterpret4/1
  reinterpret4/1 -> concatenate/4
  in5/1 -> reinterpret5/1
  reinterpret5/1 -> concatenate/5
  in6/1 -> reinterpret6/1
  reinterpret6/1 -> concatenate/6
  in7/1 -> reinterpret7/1
  reinterpret7/1 -> concatenate/7
  in8/1 -> reinterpret8/1
  reinterpret8/1 -> concatenate/8

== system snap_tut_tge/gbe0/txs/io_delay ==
  d : Inport
  Register{0..4} (5 alike) : xbsIndex_r4/Register  init=0  rst=off  en=off  dbl_ovrd=off  block_type=register
  q : Outport
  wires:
  Register0/1 -> Register1/1
  Register1/1 -> Register2/1
  Register2/1 -> Register3/1
  Register3/1 -> Register4/1
  d/1 -> Register0/1
  Register4/1 -> q/1
